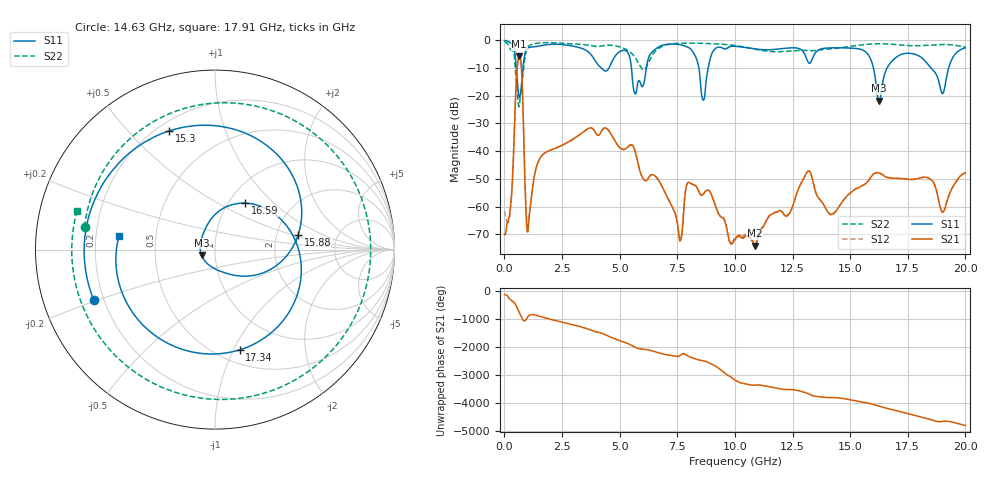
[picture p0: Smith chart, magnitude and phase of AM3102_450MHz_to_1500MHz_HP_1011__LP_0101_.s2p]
!Agilent Technologies,E8364B,MY43040894,A.07.50.67
!Agilent E8364B: A.07.50.67
!Date: Thursday, January 11, 2018 06:24:09
!Correction: S11(Full 2 Port(1,2))
!S21(Full 2 Port(1,2))
!S12(Full 2 Port(1,2))
!S22(Full 2 Port(1,2))
!S2P File: Measurements: S11, S21, S12, S22:
# Hz S  dB  R 50
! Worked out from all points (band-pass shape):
!   1601 points, 10 MHz to 20 GHz, reference 50 ohm
!   highest |S21| = -5.73 dB at 647.2 MHz (marker M1); lowest = -74.1 dB at 10.87 GHz (marker M2)
!   |S21| within 3 dB of the highest: 567.5 MHz to 728.5 MHz (161 MHz wide, 24.9 % of centre)
!   lowest |S11| = -21.8 dB at 16.25 GHz (marker M3), VSWR 1.18, Z = 42.9 - j2.62 ohm
!   |S11| at or under -10 dB: 5.514 GHz to 6.159 GHz (645.3 MHz wide, 11.1 % of centre); 16.01 GHz to 16.6 GHz (591.6 MHz wide, 3.63 % of centre); 18.5 GHz to 19.27 GHz (767.7 MHz wide, 4.06 % of centre)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
!   |S22| runs from -24.0 to -0.4 dB; largest |S21 - S12| = 0.0028
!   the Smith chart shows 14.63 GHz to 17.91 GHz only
!   S11 on the Smith chart (normalised r, x): 14.63 GHz: 0.16, -0.19; 15.3 GHz: 0.25, +0.66; 15.88 GHz: 2.64, +0.54; 16.59 GHz: 1.19, +0.68; 17.34 GHz: 0.63, -1.06; 17.91 GHz: 0.30, +0.07
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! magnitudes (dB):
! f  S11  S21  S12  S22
! 10 MHz  -0.1  -69.9  -61.6  -0.4
! 259.9 MHz  -0.9  -60.8  -61.4  -3.2
! 647.2 MHz  -20.6  -5.7  -5.7  -23.8
! 1.022 GHz  -2.7  -68.9  -66.6  -2.4
! 1.559 GHz  -2.0  -42.3  -42.3  -0.9
! 3.346 GHz  -2.9  -33.5  -33.5  -1.5
! 5.67 GHz  -19.3  -40.0  -40.0  -6.2
! 6.682 GHz  -2.4  -50.4  -50.4  -3.0
! 7.631 GHz  -1.6  -72.4  -71.6  -1.1
! 8.618 GHz  -21.6  -55.7  -55.4  -1.1
! 10.01 GHz  -2.1  -71.9  -71.4  -1.9
! 10.87 GHz  -3.1  -74.1  -74.2  -3.2
! 13.34 GHz  -7.1  -49.4  -49.3  -3.8
! 14.63 GHz  -2.7  -58.7  -58.8  -2.6
! 15.3 GHz  -3.0  -53.4  -53.3  -1.8
! 15.88 GHz  -6.6  -49.7  -49.7  -1.3
! 16.25 GHz  -21.8  -47.8  -47.9  -1.2
! 16.59 GHz  -10.2  -49.5  -49.4  -1.3
! 16.68 GHz  -8.9  -49.6  -49.6  -1.3
! 17.34 GHz  -4.8  -50.0  -50.0  -1.8
! 17.91 GHz  -5.4  -50.0  -50.0  -2.0
! 20 GHz  -2.7  -47.9  -47.8  -2.3
